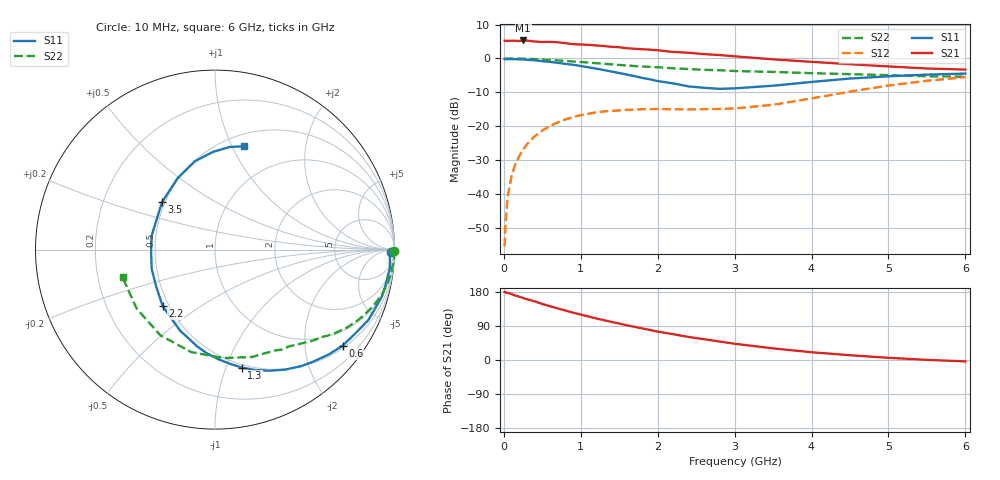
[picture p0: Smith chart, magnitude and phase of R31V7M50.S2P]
! SIEMENS Small Signal Semiconductors
! BFR181
! Si NPN RF Bipolar Junction Transistor in SOT23
! VCE = 1.75 V  IC = 0.5 mA
! Common Emitter S-Parameters:  May  1996
# GHz  S  MA  R  50
!  f  S11  S21  S12  S22
! GHz  MAG  ANG  MAG  ANG  MAG  ANG  MAG  ANG
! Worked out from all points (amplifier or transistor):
!   36 points, 10 MHz to 6 GHz, reference 50 ohm
!   highest |S21| = 5.3 dB at 250 MHz (marker M1)
!   |S21| within 3 dB of that: start of sweep to 2.041 GHz
!   unconditionally stable (mu >= 1): 2.332 GHz to 4.004 GHz
!   at 250 MHz: K = 0.13, MSG = 16.1 dB, |S12| = -26.9 dB
!   at 1.4 GHz: K = 0.62, MSG = 9.4 dB, |S12| = -15.5 dB
!   at 6 GHz: K = 0.93, MSG = 1.1 dB, |S12| = -5.5 dB
!   S11 on the Smith chart (normalised r, x): 10 MHz: 69, -51; 600 MHz: 0.56, -2.89; 1.3 GHz: 0.47, -1.14; 2.2 GHz: 0.46, -0.36; 3.5 GHz: 0.48, +0.30; 6 GHz: 0.62, +1.11
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0.01  0.9815 -0.8  1.83 179.7  0.0017 93.9  0.9996 -0.4
0.02  0.9729 -1.2  1.828 178.5  0.0034 88.2  0.9981 -0.7
0.05  0.9758 -3.0  1.815 177.0  0.0092 89.4  0.9988 -1.5
0.1  0.9797 -6.2  1.827 174.1  0.0184 86.1  0.9992 -2.9
0.15  0.974 -8.9  1.822 170.0  0.0276 82.9  0.9946 -4.5
0.25  0.9662 -15.5  1.842 163.7  0.0452 78.8  0.9912 -7.4
0.4  0.9405 -24.6  1.779 154.9  0.0708 72.8  0.9771 -11.7
0.6  0.89 -37.0  1.759 142.0  0.1011 64.8  0.9508 -17.1
0.8  0.8314 -48.5  1.681 130.5  0.126 57.3  0.9188 -22.1
1.1  0.7398 -65.8  1.588 114.9  0.1531 48.4  0.8684 -28.6
1.3  0.6741 -77.2  1.526 105.2  0.1652 43.1  0.8351 -32.5
1.6  0.578 -94.8  1.413 91.4  0.1745 37.4  0.7884 -37.5
1.8  0.515 -106.8  1.367 83.3  0.1786 35.1  0.7624 -40.4
2  0.4632 -119.8  1.319 75.0  0.1797 33.2  0.7408 -43.4
2.2  0.4287 -132.9  1.247 68.1  0.1778 32.6  0.7162 -46.6
2.4  0.3869 -147.9  1.214 60.9  0.1769 33.0  0.6976 -49.5
2.8  0.3561 -177.7  1.123 48.9  0.1797 36.0  0.671 -56.0
3.5  0.396 138.3  0.97 30.7  0.2069 45.5  0.6328 -71.0
4.5  0.5054 102.7  0.822 12.6  0.3239 48.5  0.5861 -103.2
5  0.5447 91.1  0.762 5.8  0.3983 43.4  0.566 -122.5
5.5  0.5776 81.9  0.711 0.4  0.4684 35.8  0.5465 -143.0
6  0.5977 74.4  0.685 -3.7  0.5299 27.2  0.5377 -163.4
